(* Logix 5000 DataType export Motor_Data; software revision 35.00 *)

TYPE Motor_Data :
STRUCT
   PB_Start : BOOL;
   PB_Stop : BOOL;
   Running : BOOL;
   Voltage : REAL;
   Current : REAL;
   Power : REAL;
   Overload_Trip : BOOL;
   Phase_LossTrip : BOOL;
   Ground_Fault_Current_Trip : BOOL;
   Stall_Trip : BOOL;
   Trip_Reset : BOOL;
   Load_Percent : REAL;
END_STRUCT
END_TYPE
